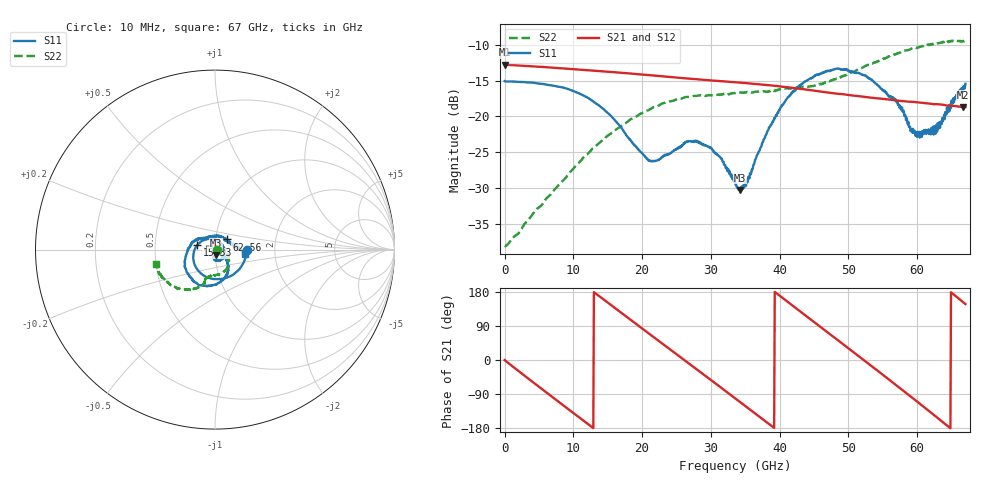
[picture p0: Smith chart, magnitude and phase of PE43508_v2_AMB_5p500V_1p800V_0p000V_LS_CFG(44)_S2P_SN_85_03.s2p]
!Keysight Technologies,N5227A,US51270237,A.10.43.00
!Date: Wednesday, August 22, 2018 17:11:10
!Correction: S11(Full 2 Port(1,3))
!S31(Full 2 Port(1,3))
!S13(Full 2 Port(1,3))
!S33(Full 2 Port(1,3))
!S2P File: Measurements: S11, S31, S13, S33:
# Hz S  dB  R 50
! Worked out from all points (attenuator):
!   801 points, 10 MHz to 67 GHz, reference 50 ohm
!   highest |S21| = -12.73 dB at 10 MHz (marker M1); lowest = -18.7 dB at 66.67 GHz (marker M2)
!   lowest |S11| = -30.3 dB at 34.17 GHz (marker M3), VSWR 1.06, Z = 50.4 - j3.04 ohm
!   |S11| at or under -10 dB: start of sweep to end of sweep
!   |S22| runs from -38.2 to -9.4 dB; largest |S21 - S12| = 0.0011
!   S11 on the Smith chart (normalised r, x): 10 MHz: 1.43, -0.00; 15.33 GHz: 0.82, +0.04; 62.56 GHz: 1.13, +0.13; 67 GHz: 1.40, -0.07
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1e7  -15.05 -0.4  -12.73 -0.2  -12.73 -0.2  -38.13 -1.0
5.70415e9  -15.47 -75.0  -13.08 -80.5  -13.09 -80.4  -32.02 15.2
8.300012e9  -15.91 -106.9  -13.26 -116.4  -13.26 -116.4  -29.16 10.1
1.123082e10  -16.95 -141.9  -13.46 -156.7  -13.46 -156.7  -26.03 -2.4
1.533396e10  -19.79 165.9  -13.76 147.0  -13.76 147.0  -22.47 -20.4
1.885094e10  -24.04 106.1  -14.04 98.9  -14.03 98.9  -20.16 -37.2
2.102811e10  -26.13 56.0  -14.22 69.2  -14.22 69.2  -19.08 -48.3
2.236791e10  -26.10 20.5  -14.33 51.0  -14.33 51.0  -18.47 -54.8
2.521499e10  -24.52 -34.2  -14.57 12.3  -14.57 12.3  -17.57 -67.4
2.797832e10  -23.56 -68.0  -14.79 -25.2  -14.80 -25.2  -17.12 -78.1
3.124409e10  -25.59 -96.0  -15.05 -69.6  -15.05 -69.5  -16.98 -88.2
3.3505e10  -29.22 -90.1  -15.21 -100.6  -15.21 -100.6  -16.73 -93.3
3.41749e10  -30.31 -80.4  -15.26 -109.7  -15.27 -109.7  -16.64 -94.4
3.526349e10  -28.82 -54.6  -15.34 -124.8  -15.35 -124.7  -16.57 -95.7
4.0204e10  -18.64 -51.0  -15.81 166.8  -15.81 166.9  -16.15 -103.3
4.472582e10  -14.58 -84.3  -16.34 104.0  -16.33 104.1  -15.76 -106.5
4.975008e10  -13.52 -124.8  -16.97 34.3  -16.96 34.3  -14.20 -108.2
5.586291e10  -17.24 171.7  -17.61 -51.4  -17.60 -51.7  -11.59 -122.2
5.96311e10  -22.00 108.2  -18.00 -104.7  -18.01 -104.9  -10.45 -134.3
6.256191e10  -21.36 41.3  -18.28 -146.9  -18.31 -147.2  -9.80 -146.7
6.666505e10  -16.40 -5.2  -18.70 152.6  -18.76 152.6  -9.41 -164.2
6.7e10  -15.43 -7.9  -18.70 147.6  -18.76 147.6  -9.40 -166.3
